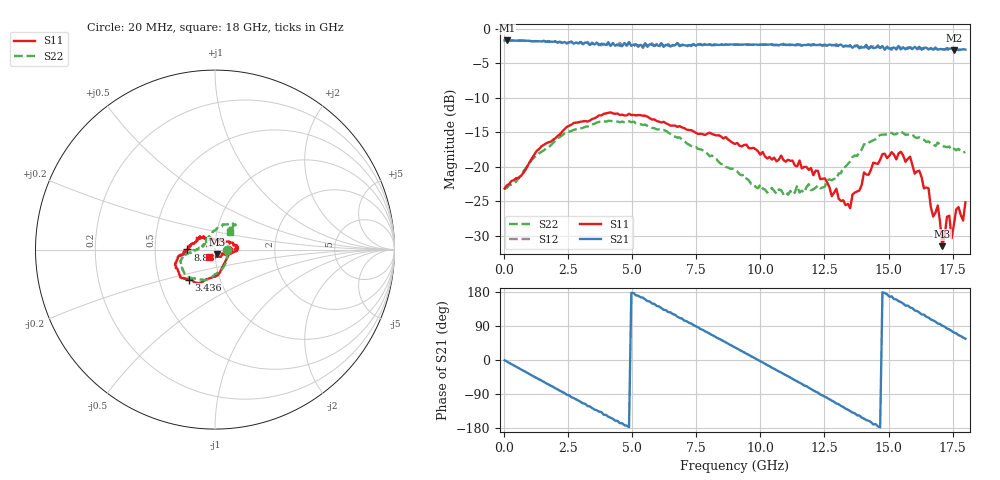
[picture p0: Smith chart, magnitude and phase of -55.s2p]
!Agilent Technologies,N5230A,US43500223,A.07.50.48
!Agilent N5230A: A.07.50.48
!Date: Sunday, January 17, 2016 17:51:39
!Correction: S11(Full 2 Port(1,2))
!S21(Full 2 Port(1,2))
!S12(Full 2 Port(1,2))
!S22(Full 2 Port(1,2))
!S2P File: Measurements: S11, S21, S12, S22:
# Hz S  RI  R 50
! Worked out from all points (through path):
!   201 points, 20 MHz to 18 GHz, reference 50 ohm
!   highest |S21| = -1.70 dB at 109.9 MHz (marker M1); lowest = -3.1 dB at 17.55 GHz (marker M2)
!   group delay of S21, straight-line fit = 102 ps
!   lowest |S11| = -31.5 dB at 17.1 GHz (marker M3), VSWR 1.05, Z = 50.9 - j2.53 ohm
!   |S11| at or under -10 dB: start of sweep to end of sweep
!   |S22| runs from -24.0 to -13.3 dB; largest |S21 - S12| = 0.054
!   S11 on the Smith chart (normalised r, x): 20 MHz: 1.15, -0.01; 3.436 GHz: 0.71, -0.25; 8.83 GHz: 0.73, +0.00; 18 GHz: 0.93, -0.08
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2e7  0.0697 -0.00318  0.8217 -0.0114  0.8219 -0.0122  0.069 -0.0035
1.099e8  0.0724 -0.0134  0.8197 -0.0595  0.8201 -0.0604  0.0696 -0.0126
1.7281e9  0.00145 -0.1504  0.3493 -0.7241  0.3507 -0.7343  -0.00151 -0.1382
3.0766e9  -0.1104 -0.1825  -0.3201 -0.7029  -0.3244 -0.7087  -0.1033 -0.1615
3.4362e9  -0.1466 -0.1668  -0.4768 -0.633  -0.4747 -0.6252  -0.1247 -0.1605
4.8746e9  -0.219 -0.1034  -0.8012 -0.0367  -0.7829 -0.0424  -0.19 -0.0975
6.0433e9  -0.2074 -0.0463  -0.5886 0.468  -0.559 0.4761  -0.1816 -0.0432
7.3918e9  -0.1784 -0.0273  -0.0284 0.7737  -0.0294 0.7715  -0.139 -0.0148
8.8302e9  -0.1533 0.000724  0.5922 0.4927  0.5992 0.4762  -0.0967 0.00456
9.01e9  -0.1464 0.00305  0.6422 0.4207  0.6502 0.4059  -0.0952 0.00218
1.04484e10  -0.1026 0.047  0.7227 -0.2666  0.7123 -0.2846  -0.0633 0.0307
1.20666e10  -0.061 0.062  0.1346 -0.7622  0.1151 -0.7532  -0.0411 0.0552
1.3505e10  0.0229 0.0446  -0.5337 -0.5399  -0.5331 -0.52  0.00517 0.1093
1.40444e10  0.0791 0.0457  -0.6614 -0.3114  -0.6711 -0.2885  0.0425 0.1396
1.50333e10  0.1183 0.023  -0.6974 0.1609  -0.7006 0.1766  0.1013 0.1453
1.6202e10  0.0919 -0.0191  -0.4292 0.6046  -0.3938 0.5977  0.1039 0.1265
1.67414e10  0.0381 -0.0215  -0.1765 0.6827  -0.1476 0.6938  0.0852 0.1175
1.69212e10  0.0327 -0.0411  -0.0765 0.7009  -0.055 0.7059  0.0875 0.1218
1.7101e10  0.00978 -0.0248  -0.000467 0.7111  0.023 0.7104  0.0783 0.1183
1.72808e10  0.00289 -0.0435  0.0826 0.7196  0.1085 0.7  0.0781 0.1149
1.75505e10  -0.00542 -0.0377  0.2105 0.6677  0.2331 0.6615  0.0802 0.1092
1.8e10  -0.0351 -0.0429  0.3928 0.5874  0.4194 0.5633  0.0822 0.0987
